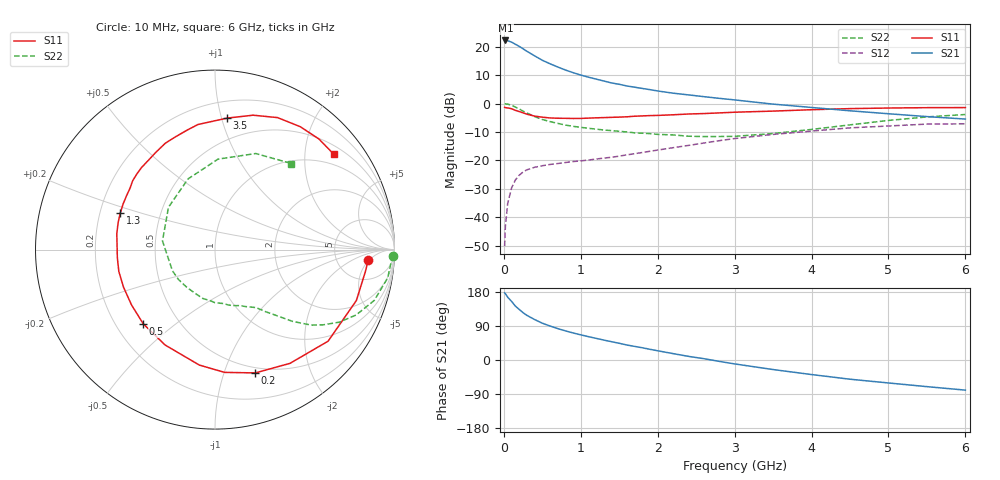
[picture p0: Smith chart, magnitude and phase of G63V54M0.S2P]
! SIEMENS Small Signal Semiconductors
! BFG193
! Si NPN RF Bipolar Junction Transistor in SOT223
! VCE = 3.5 V  IC = 4 mA
! Common Emitter S-Parameters:  August  1996
# GHz  S  MA  R  50
!  f  S11  S21  S12  S22
! GHz  MAG  ANG  MAG  ANG  MAG  ANG  MAG  ANG
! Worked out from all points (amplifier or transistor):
!   36 points, 10 MHz to 6 GHz, reference 50 ohm
!   highest |S21| = 22.2 dB at 20 MHz (marker M1)
!   |S21| within 3 dB of that: start of sweep to 253.9 MHz
!   unconditionally stable (mu >= 1): 1.194 GHz to 2.56 GHz
!   at 250 MHz: K = 0.29, MSG = 21.7 dB, |S12| = -24.1 dB
!   at 1.4 GHz: K = 1.09, MAG = 11.3 dB, |S12| = -18.9 dB
!   at 6 GHz: K = 0.89, MSG = 0.8 dB, |S12| = -7.1 dB
!   S11 on the Smith chart (normalised r, x): 10 MHz: 11, -5; 200 MHz: 0.44, -1.28; 500 MHz: 0.31, -0.39; 1.3 GHz: 0.29, +0.17; 3.5 GHz: 0.33, +1.04; 6 GHz: 0.70, +2.68
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0.01  0.8552 -4.0  12.85 177.1  0.0031 90.4  0.9925 -1.9
0.02  0.8471 -8.2  12.86 175.1  0.0069 86.0  0.9847 -3.7
0.05  0.8372 -19.8  12.7 165.8  0.0175 78.9  0.9751 -9.3
0.1  0.8108 -39.0  12.03 154.7  0.0326 71.2  0.9315 -17.7
0.15  0.7591 -56.6  11.04 142.2  0.0453 61.9  0.8662 -24.9
0.2  0.7228 -71.9  10.13 133.4  0.0549 55.8  0.8015 -30.3
0.25  0.6862 -85.5  9.175 124.8  0.0625 49.9  0.7344 -34.8
0.3  0.6493 -97.7  8.294 117.8  0.0683 46.0  0.682 -38.1
0.4  0.5999 -117.6  6.89 106.8  0.0756 40.4  0.5884 -42.8
0.5  0.5752 -134.0  5.767 97.1  0.0805 36.6  0.5241 -45.8
0.6  0.558 -146.5  5 89.7  0.0848 34.6  0.4813 -48.3
0.7  0.551 -157.7  4.396 82.9  0.088 34.0  0.448 -50.7
0.9  0.5459 -175.4  3.491 71.4  0.0954 33.5  0.3973 -54.6
1.1  0.5542 170.8  2.905 61.6  0.1015 34.2  0.3669 -60.3
1.3  0.5656 159.1  2.489 52.6  0.1098 35.1  0.3421 -65.7
1.6  0.5842 144.1  2.036 39.5  0.1251 35.4  0.3163 -76.9
2.2  0.6337 121.5  1.521 16.9  0.1672 33.2  0.2804 -104.3
2.8  0.684 103.0  1.233 -3.6  0.2222 25.5  0.263 -140.6
3.5  0.7358 84.7  0.976 -25.2  0.2862 11.1  0.2966 170.6
4.5  0.814 64.6  0.745 -50.7  0.3734 -10.2  0.4214 110.9
5.5  0.8456 46.8  0.589 -70.3  0.4346 -36.8  0.5815 67.0
6  0.8486 38.8  0.533 -79.5  0.4403 -51.8  0.6413 48.4
